TYPE DUT_AMCI_Stepper :
STRUCT
  //Network Address
	sNetId				: T_AmsNetId;
	nSlaveAddr			: UINT;
  //Outputs:
	nCMD0 AT %Q* 		: UINT;	
	nCMD1 AT %Q* 		: UINT := 16#8000;
	nTargetPos AT %Q* 	: DINT;
	nTargetVel AT %Q* 	: UDINT;
	nAccel AT %Q* 		: UINT;
	nDecel AT %Q* 		: UINT;
	nMtr_Curr AT %Q*	: UINT;
	nJerk AT %Q* 		: UINT := 0;
  //Inputs:
	iStatus0 AT %I* 	: UINT;
	iStatus1 AT %I* 	: UINT;
	iMotorPos AT %I* 	: DINT;
	iEncPos AT %I* 		: DINT;
	iTrapped_enc AT %I* : DINT;
	iMtr_Current AT %I* : UINT;
	iJerk AT %I* 		: UINT;
END_STRUCT
END_TYPE
